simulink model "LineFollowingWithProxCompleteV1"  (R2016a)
settings: Solver=VariableStepDiscrete  StartTime=0.0  StopTime=inf  RelTol=1e-3
model workspace (MAT data in the model file):
  MCOS : class17 (value not decoded)
  MCOS : class17 (value not decoded)
  MCOS : class17 (value not decoded)
  MCOS : class17 (value not decoded)
  MCOS : class17 (value not decoded)
  MCOS : class17 (value not decoded)
undefined symbols (not defined in the file or in its folder): axleLength, commandPercmPerSecond, symmetrizeMotors
libraries: miniQ x3, simulink x1

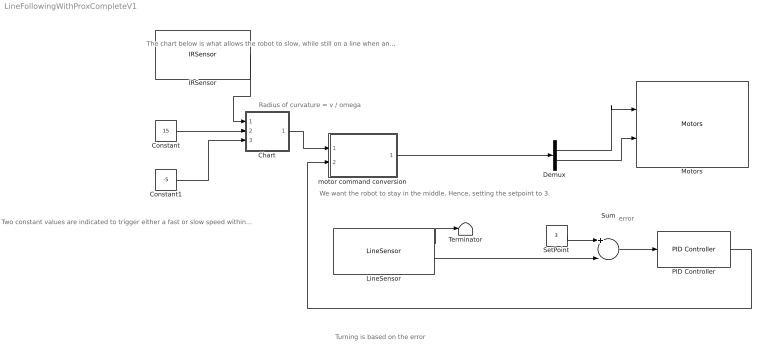
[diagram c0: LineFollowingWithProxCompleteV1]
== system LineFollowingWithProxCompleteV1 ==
  note: Two constant values are indicated to trigger either a fast or slow speed within the chart
  note: The chart below is what allows the robot to slow, while still on a line when an object is infront of it. Click into the chart to view how.
  note: Turning is based on the error
  note: error
  note: We want the robot to stay in the middle. Hence, setting the setpoint to 3.
  note: Radius of curvature = v / omega
  Chart : Stateflow chart  TreatAsAtomicUnit=on
  Constant : Constant  Value=15
  Constant1 : Constant  Value=-5
  Demux : Demux  Outputs=2
  IRSensor : miniQ/IRSensor  sampleTime_dd=0.01  debug_dd=off
  LineSensor : miniQ/LineSensor  sampleTime_dd=0.01  maxRawSensors=[983,813,642,917,813]  minRawSensors=[703,343,250,439,368]  debug_dd=off
  Motors : miniQ/Motors  flipLeft=off  flipRight=off
  PID Controller : simulink/Continuous/PID Controller  Controller=PID  TimeDomain=Discrete-time  SampleTime=-1  IntegratorMethod=Forward Euler  FilterMethod=Forward Euler  Form=Parallel  UseFilter=on  ControllerParametersSource=internal  P=10  I=0  D=0.005  N=1  InitialConditionSource=internal  InitialConditionForIntegrator=0  InitialConditionForFilter=0  ExternalReset=none  LimitOutput=off  UpperSaturationLimit=5  LowerSaturationLimit=-5  LinearizeAsGain=on  AntiWindupMode=none  Kb=1  TrackingMode=off  Kt=1  PParamMin=[]  PParamMax=[]  IParamMin=[]  IParamMax=[]  DParamMin=[]  DParamMax=[]  NParamMin=[]  NParamMax=[]  KbParamMin=[]  KbParamMax=[]  KtParamMin=[]  KtParamMax=[]  POutMin=[]  POutMax=[]  IOutMin=[]  IOutMax=[]  DOutMin=[]  DOutMax=[]  NOutMin=[]  NOutMax=[]  KbOutMin=[]  KbOutMax=[]  KtOutMin=[]  KtOutMax=[]  IntegratorOutMin=[]  IntegratorOutMax=[]  FilterOutMin=[]  FilterOutMax=[]  SumOutMin=[]  SumOutMax=[]  SumI1OutMin=[]  SumI1OutMax=[]  SumI2OutMin=[]  SumI2OutMax=[]  SumI3OutMin=[]  SumI3OutMax=[]  SumDOutMin=[]  SumDOutMax=[]  SaturationOutMin=[]  SaturationOutMax=[]  IntegratorContinuousStateAttributes=''  IntegratorStateMustResolveToSignalObject=off  IntegratorRTWStateStorageClass=Auto  FilterContinuousStateAttributes=''  FilterStateMustResolveToSignalObject=off  FilterRTWStateStorageClass=Auto  DifferentiatorICPrevScaledInput=0  DifferentiatorOutMin=[]  DifferentiatorOutMax=[]
  SetPoint : Constant  Value=3
  Sum : Sum  Inputs=+-
  Terminator : Terminator
  motor command conversion : Subsystem
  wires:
  motor command conversion/1(v_L v_R) -> Demux/1
  LineSensor/1 -> Terminator/1
  LineSensor/2 -> Sum/2
  SetPoint/1 -> Sum/1
  Sum/1 -> PID Controller/1
  PID Controller/1 -> motor command conversion/2(omega)
  Demux/1 -> Motors/1
  Demux/2 -> Motors/2
  Chart/1(v) -> motor command conversion/1(v)
  IRSensor/1 -> Chart/1(prox)
  Constant1/1 -> Chart/3(slow)
  Constant/1 -> Chart/2(fast)

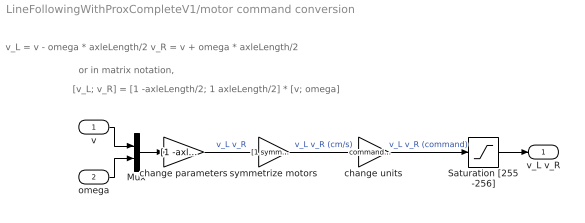
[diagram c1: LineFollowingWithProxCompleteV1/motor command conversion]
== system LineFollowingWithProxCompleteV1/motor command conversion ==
  note: or in matrix notation,
  note: v_L = v - omega * axleLength/2 v_R = v + omega * axleLength/2
  note: [v_L; v_R] = [1 -axleLength/2; 1 axleLength/2] * [v; omega]
  v : Inport
  omega : Inport  Port=2
  Mux : Mux  Inputs=2
  Saturation [255 -256] : Saturate  UpperLimit=255  LowerLimit=-256
  change parameters : Gain  Gain=[1 -axleLength/2; 1 axleLength/2]  Multiplication=Matrix(K*u)
  change units : Gain  Gain=commandPercmPerSecond
  symmetrize motors : Gain  Gain=[1 symmetrizeMotors]
  v_L v_R : Outport
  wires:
  change parameters/1 -> symmetrize motors/1  "v_L v_R"
  change units/1 -> Saturation [255 -256]/1  "v_L v_R (command)"
  symmetrize motors/1 -> change units/1  "v_L v_R (cm/s)"
  Saturation [255 -256]/1 -> v_L v_R/1
  Mux/1 -> change parameters/1
  omega/1 -> Mux/2
  v/1 -> Mux/1

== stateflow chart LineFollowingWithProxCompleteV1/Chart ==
  state Go
    entry: v=fast
  state If an object is infront of the robot then v is set to the "slow" value, -5 [group]
  state Stop
    entry: v=slow
  state Without the object, [group]
    v is set to the "fast" value,
    15
  (default) -> Go
  Go -> Stop : [prox>10]
  Stop -> Go : [prox<10]
  data: prox input; v output; fast input; slow input
